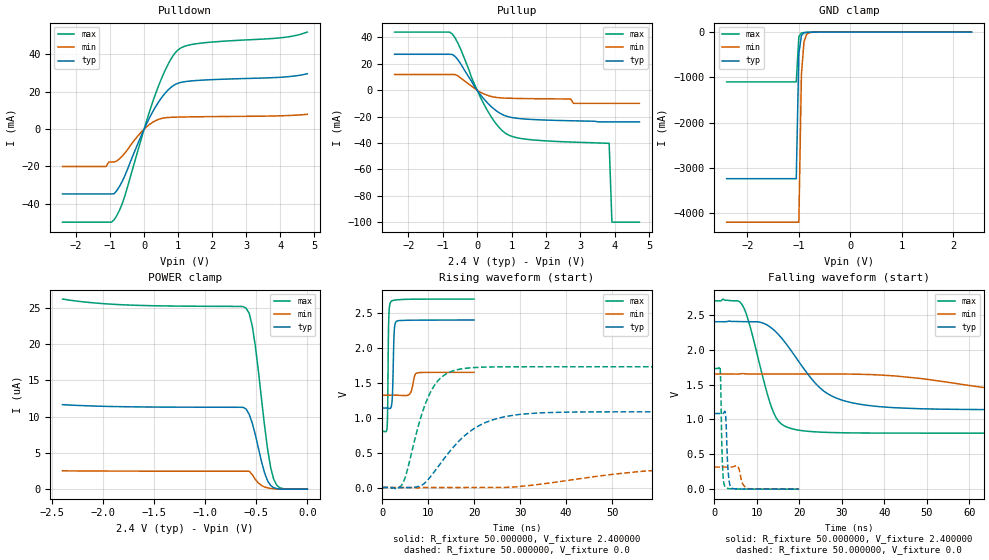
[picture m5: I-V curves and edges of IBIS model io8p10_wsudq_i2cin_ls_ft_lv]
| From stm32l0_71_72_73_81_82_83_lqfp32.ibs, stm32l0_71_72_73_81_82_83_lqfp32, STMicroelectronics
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|   Model io8p10_wsudq_i2cin_ls_ft_lv
[Model]  io8p10_wsudq_i2cin_ls_ft_lv
Model_type I/O
Polarity   Non-Inverting
Enable   Active-Low
Vinl =   0.720000V
Vinh =   1.680000V
Vmeas =  1.200000V
Cref =   50.000000pF
Rref =   100.000000M
Vref =   0.0V
C_comp   2.943600pF   2.919700pF   2.965100pF
[Temperature Range]   25.000000   0.105000k   -40.000000
[Pullup Reference]   2.400000V   1.650000V   2.700000V
[Pulldown Reference]   0.0V   0.0V   0.0V
[POWER Clamp Reference]   2.400000V   1.650000V   2.700000V
[GND Clamp Reference]   0.0V   0.0V   0.0V
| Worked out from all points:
|   slope of the pulldown table from 0 to 0.36 V, typ, clamps not added: 28.5 ohm
|   slope of the pullup table from 0 to 0.36 V, typ, clamps not added: 32.2 ohm
|   GND clamp passes 1 mA (typ) near -0.65 V on its own axis
|   rising waveform, R_fixture 50.000000, V_fixture 2.400000: 20-80 % time 286ps typ, 638ps min, 195ps max; typ from 1.14 V to 2.4 V
|   rising waveform, R_fixture 50.000000, V_fixture 0.0: 20-80 % time 9.34ns typ, 24.6ns min, 4.83ns max; typ from 0 V to 1.08 V
|   falling waveform, R_fixture 50.000000, V_fixture 2.400000: 20-80 % time 10ns typ, 27ns min, 4.95ns max; typ from 2.4 V to 1.14 V
|   falling waveform, R_fixture 50.000000, V_fixture 0.0: 20-80 % time 484ps typ, 855ps min, 381ps max; typ from 1.08 V to 0 V
[Pulldown]
|Voltage   I(typ)   I(min)   I(max)
-2.4V     -34.71mA   -20mA      -49.82mA
-1.12V    -34.71mA   -20mA      -49.82mA
-1.04V    -34.71mA   -17.6mA    -49.82mA
-880mV    -34.55mA   -17.6mA    -48.46mA
-560mV    -24.65mA   -12.68mA   -35.33mA
0V        225fA      0A         140fA
400mV     13.84mA    5.066mA    22.03mA
720mV     21.25mA    6.254mA    35.26mA
1.04V     24.82mA    6.464mA    43.03mA
1.6V      26.11mA    6.627mA    45.88mA
4V        27.76mA    7.125mA    48.87mA
4.8V      29.64mA    7.94mA     51.96mA
[Pullup]
|Voltage   I(typ)   I(min)   I(max)
-2.4V     27.21mA    11.89mA    44.01mA
-720mV    27.06mA    11.89mA    42.53mA
-480mV    20.06mA    9.352mA    31.11mA
-160mV    6.586mA    3.048mA    9.467mA
240mV     -7.917mA   -3.299mA   -12.65mA
560mV     -15.67mA   -5.497mA   -25.76mA
880mV     -19.92mA   -6.062mA   -33.51mA
1.68V     -22.29mA   -6.449mA   -37.81mA
2.8V      -23.2mA    -10mA      -39.35mA
3.84V     -24mA      -10mA      -40.2mA
3.92V     -24mA      -10mA      -100mA
4.72V     -24mA      -10mA      -100mA
[GND_clamp]
|Voltage   I(typ)   I(min)   I(max)
-2.4V     -3.237A    -4.198A    -1.1A
-1.05V    -3.237A    -4.198A    -1.1A
-1V       -475.8mA   -4.198A    -104.2mA
-950mV    -76.24mA   -935.4mA   -18.39mA
-900mV    -16.61mA   -212.9mA   -9.105mA
-850mV    -6.547mA   -50.94mA   -6.589mA
-800mV    -3.998mA   -13.81mA   -4.86mA
-650mV    -1.043mA   -1.182mA   -1.146mA
2.35V     0A         0A         0A
[POWER_clamp]
|Voltage   I(typ)   I(min)   I(max)
-2.4V     11.64uA    2.525uA    26.17uA
-1.86V    11.37uA    2.488uA    25.42uA
-600mV    11.04uA    2.474uA    24.9uA
-570mV    10.3uA     2.473uA    24.21uA
-540mV    9.097uA    2uA        22.48uA
-510mV    7.497uA    1.35uA     19.73uA
-450mV    3.845uA    512.5nA    12.52uA
-390mV    1.154uA    175.5nA    5.528uA
-360mV    508.2nA    102.8nA    2.997uA
-330mV    204.4nA    60.39nA    1.375uA
-270mV    0A         0A         194.9nA
0V        0A         0A         0A
[Ramp]
| variable   typ   min   max
dV/dt_r  0.65070/9.33339n   0.18997/24.62510n   1.03800/4.81953n
dV/dt_f  0.75690/10.02985n   0.19674/26.99226n   1.13815/4.93620n
R_load = 50.000000
[Rising Waveform]
R_fixture= 50.000000
V_fixture= 2.400000
V_fixture_min= 1.650000
V_fixture_max= 2.700000
|time   V(typ)   V(min)   V(max)
0s        1.139V     1.322V     803.1mV
1.041ns   1.138V     1.322V     868.1mV
1.161ns   1.137V     1.322V     1.18V
1.401ns   1.134V     1.322V     2.435V
1.842ns   1.143V     1.322V     2.661V
2.202ns   1.336V     1.322V     2.678V
2.603ns   2.258V     1.322V     2.684V
3.003ns   2.377V     1.322V     2.688V
7.528ns   2.398V     1.64V      2.699V
19.94ns   2.4V       1.65V      2.7V
[Rising Waveform]
R_fixture= 50.000000
V_fixture= 0.0
V_fixture_min= 0.0
V_fixture_max= 0.0
|time   V(typ)   V(min)   V(max)
0s        -519nV     -2.974uV   -280.6nV
4.505ns   -925.2uV   97.58uV    65.32mV
8.509ns   31.91mV    -956uV     1.034V
11.51ns   243.2mV    -199.9uV   1.481V
14.01ns   463.1mV    -201uV     1.632V
18.02ns   748.3mV    -177.5uV   1.707V
26.53ns   1.013V     1.744mV    1.729V
40.54ns   1.081V     103.2mV    1.73V
80.08ns   1.085V     302.3mV    1.73V
249.2ns   1.085V     316.6mV    1.73V
[Falling Waveform]
R_fixture= 50.000000
V_fixture= 2.400000
V_fixture_min= 1.650000
V_fixture_max= 2.700000
|time   V(typ)   V(min)   V(max)
0s        2.4V       1.65V      2.7V
6.507ns   2.401V     1.657V     2.646V
8.008ns   2.4V       1.651V     2.414V
14.01ns   2.281V     1.65V      1.086V
16.52ns   2.113V     1.65V      905.3mV
21.02ns   1.73V      1.65V      835.6mV
28.53ns   1.31V      1.65V      810.3mV
42.54ns   1.167V     1.623V     803.6mV
91.09ns   1.139V     1.351V     803.1mV
249.2ns   1.139V     1.322V     803.1mV
[Falling Waveform]
R_fixture= 50.000000
V_fixture= 0.0
V_fixture_min= 0.0
V_fixture_max= 0.0
|time   V(typ)   V(min)   V(max)
0s        1.085V     316.6mV    1.73V
1.321ns   1.085V     316.6mV    1.745V
1.441ns   1.085V     316.6mV    1.593V
1.722ns   1.084V     316.6mV    682.1mV
1.922ns   1.084V     316.6mV    309.1mV
2.523ns   1.108V     316.6mV    34.21mV
3.243ns   241.8mV    316.4mV    9.332mV
3.964ns   19.96mV    316.5mV    5.619mV
7.928ns   1.336mV    8.838mV    1.293mV
19.94ns   -519nV     -2.974uV   -280.6nV
